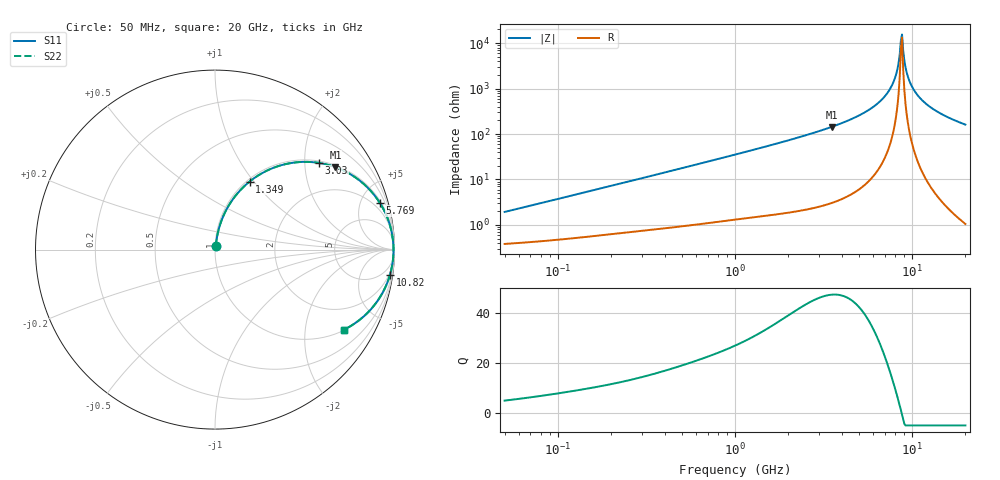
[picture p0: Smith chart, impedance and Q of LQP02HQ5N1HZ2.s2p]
!Murata Part Number: LQP02HQ5N1HZ2
!These Parameters are Measured in Series Mode Connection
!  o--[Z]--o
!Port1  Port2
!  o-------o
!Freq. Start=50[MHz] Stop=20[GHz], 401[Steps]
# Hz S RI R 50
!Freq.(Hz) S11(Real) S11(Imag) S21(Real) S21(Imag) S12(Real) S12(Imag) S22(Real) S22(Imag)
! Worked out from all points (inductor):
!   401 points, 50 MHz to 20 GHz, reference 50 ohm
!   read as one part in series: L = 5.96 nH near 51.52 MHz
!   highest Q = 47.4 at 3.519 GHz (marker M1), where L = 6.5 nH
!   self-resonance near 8.645 GHz
!   S11 on the Smith chart (normalised r, x): 50 MHz: 1.01, +0.04; 1.349 GHz: 1.03, +0.95; 3.03 GHz: 1.05, +2.36; 5.769 GHz: 1.19, +7.00; 10.82 GHz: 1, -14; 20 GHz: 1.02, -3.22
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5e7  0.00414 0.0187  0.9959 -0.0187  0.9959 -0.0187  0.00414 0.0187
1.364002e8  0.00772 0.0492  0.9923 -0.0492  0.9923 -0.0492  0.00772 0.0492
3.721004e8  0.0248 0.1277  0.9752 -0.1277  0.9752 -0.1277  0.0248 0.1277
1e9  0.1188 0.3056  0.8812 -0.3056  0.8812 -0.3056  0.1188 0.3056
1.349283e9  0.193 0.3792  0.807 -0.3792  0.807 -0.3792  0.193 0.3792
2.728004e9  0.5174 0.4887  0.4826 -0.4887  0.4826 -0.4887  0.5174 0.4887
3.029571e9  0.5802 0.4828  0.4198 -0.4828  0.4198 -0.4828  0.5802 0.4828
3.519108e9  0.6708 0.4595  0.3292 -0.4595  0.3292 -0.4595  0.6708 0.4595
5.769027e9  0.9184 0.2603  0.0816 -0.2603  0.0816 -0.2603  0.9184 0.2603
6.701223e9  0.9627 0.1715  0.0373 -0.1715  0.0373 -0.1715  0.9627 0.1715
7.442007e9  0.9826 0.105  0.0174 -0.105  0.0174 -0.105  0.9826 0.105
8.020766e9  0.991 0.0561  0.00901 -0.0561  0.00901 -0.0561  0.991 0.0561
8.264682e9  0.993 0.0364  0.00704 -0.0364  0.00704 -0.0364  0.993 0.0364
8.516016e9  0.9941 0.0166  0.00587 -0.0166  0.00587 -0.0166  0.9941 0.0166
8.774992e9  0.9945 -0.00329  0.0055 0.00329  0.0055 0.00329  0.9945 -0.00329
8.907419e9  0.9944 -0.0132  0.00561 0.0132  0.00561 0.0132  0.9944 -0.0132
9.316812e9  0.9929 -0.043  0.00714 0.043  0.00714 0.043  0.9929 -0.043
9.600142e9  0.9908 -0.0627  0.00916 0.0627  0.00916 0.0627  0.9908 -0.0627
1.004137e10  0.9863 -0.0922  0.0137 0.0922  0.0137 0.0922  0.9863 -0.0922
1.082228e10  0.9748 -0.1407  0.0252 0.1407  0.0252 0.1407  0.9748 -0.1407
1.375312e10  0.9064 -0.2844  0.0936 0.2844  0.0936 0.2844  0.9064 -0.2844
2e10  0.7201 -0.4457  0.2799 0.4457  0.2799 0.4457  0.7201 -0.4457
